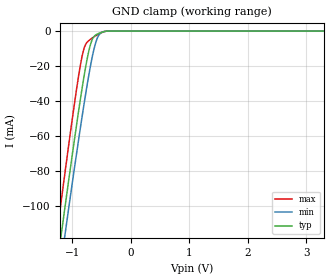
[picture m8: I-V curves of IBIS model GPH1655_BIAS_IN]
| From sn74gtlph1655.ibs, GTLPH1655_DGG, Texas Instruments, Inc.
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[Model]   GPH1655_BIAS_IN
Model_type  Input
Vinl=0.8
Vinh=2.0
| variable   typ   min   max
C_comp   8.40pF   6.26pF   11.51pF
[Temperature Range]   40   100   -40
| Ambient temperature   25   85   -40
[Voltage range]   3.3   3.15   3.45
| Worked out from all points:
|   GND clamp passes 1 mA (typ) near -0.52 V on its own axis
[GND Clamp]
| GPH1655_BIAS_IN
|   Voltage   I(typ)   I(min)   I(max)
-5.5V     -1.245A    -1.236A    -1.263A
-1.29V    -142.3mA   -157.3mA   -123.9mA
-1.25V    -132.4mA   -147.6mA   -113.5mA
-1.175V   -113.8mA   -129.4mA   -94.38mA
-1.11V    -97.86mA   -113.7mA   -77.98mA
-915mV    -51.59mA   -68.03mA   -31.18mA
-810mV    -28.64mA   -44.69mA   -11.51mA
-735mV    -14.53mA   -29.13mA   -6.08mA
-675mV    -6.474mA   -17.92mA   -4.424mA
-590mV    -2.083mA   -5.867mA   -2.527mA
-515mV    -920.2uA   -1.202mA   -1.164mA
3.3V      605.5pA    1.305nA    2.391nA
